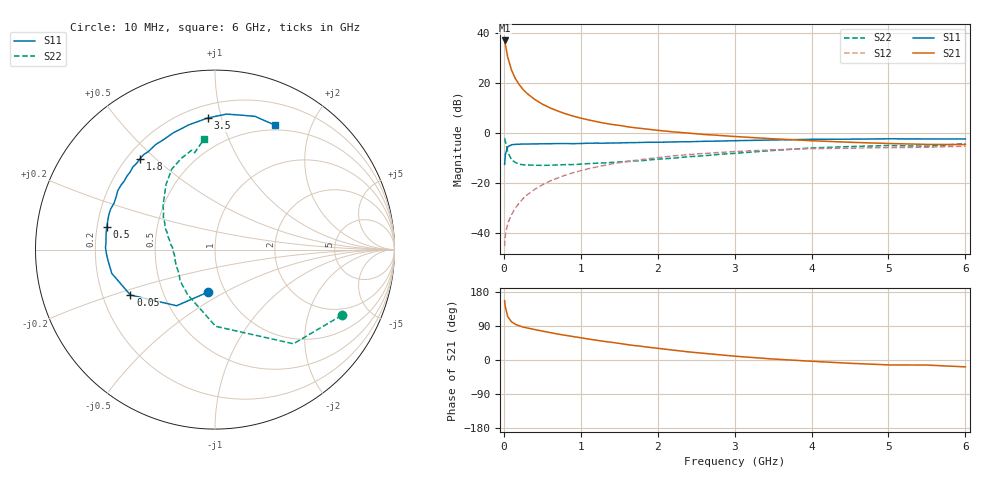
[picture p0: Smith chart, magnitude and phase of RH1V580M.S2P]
! SIEMENS Small Signal Semiconductors
! BFR106
! Si NPN RF Bipolar Junction Transistor in SOT23
! VCE = 1.5 V  IC = 80 mA
! Common Emitter S-Parameters:  August  1996
# GHz  S  MA  R  50
!  f  S11  S21  S12  S22
! GHz  MAG  ANG  MAG  ANG  MAG  ANG  MAG  ANG
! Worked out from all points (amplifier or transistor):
!   36 points, 10 MHz to 6 GHz, reference 50 ohm
!   highest |S21| = 37.2 dB at 10 MHz (marker M1)
!   |S21| within 3 dB of that: start of sweep to 27.98 MHz
!   unconditionally stable (mu >= 1): 141.1 MHz to end of sweep
!   at 250 MHz: K = 1.08, MAG = 20.1 dB, |S12| = -26.1 dB
!   at 1.4 GHz: K = 1.09, MAG = 6.1 dB, |S12| = -12.3 dB
!   at 6 GHz: K = 1.02, MAG = -0.6 dB, |S12| = -5.2 dB
!   S11 on the Smith chart (normalised r, x): 10 MHz: 0.83, -0.42; 50 MHz: 0.32, -0.23; 500 MHz: 0.24, +0.10; 1.8 GHz: 0.25, +0.45; 3.5 GHz: 0.28, +0.91; 6 GHz: 0.44, +1.51
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0.01  0.2388 -98.9  72.15 156.7  0.0055 73.3  0.7956 -27.4
0.02  0.3791 -124.4  59.42 139.6  0.0094 63.6  0.6829 -50.2
0.05  0.535 -151.8  33.65 114.7  0.0156 57.4  0.4275 -89.5
0.1  0.5901 -167.0  18.35 100.7  0.0236 64.0  0.2936 -121.3
0.15  0.5995 -174.3  12.41 94.3  0.0319 67.5  0.2613 -137.9
0.2  0.6055 -177.9  9.421 90.2  0.0404 70.3  0.24 -147.3
0.25  0.6102 178.9  7.528 87.0  0.0494 71.2  0.2345 -155.0
0.3  0.6087 176.4  6.306 84.7  0.058 72.0  0.2325 -159.2
0.4  0.6131 171.9  4.778 80.4  0.0755 72.4  0.2293 -166.3
0.5  0.6157 168.4  3.836 76.3  0.0928 71.8  0.2279 -171.2
0.6  0.6187 164.9  3.226 72.4  0.1107 70.7  0.2292 -174.2
0.7  0.6227 161.8  2.793 68.5  0.1276 69.7  0.2328 -177.0
0.9  0.619 155.3  2.21 61.9  0.1622 66.5  0.2366 177.4
1.1  0.6332 148.9  1.853 55.3  0.1952 63.2  0.2471 173.8
1.4  0.6387 140.4  1.507 46.7  0.2425 57.6  0.2606 167.8
1.8  0.6568 129.4  1.243 35.9  0.2996 50.4  0.2841 160.0
2.2  0.672 119.5  1.068 26.1  0.3515 43.2  0.3173 152.0
2.8  0.6986 105.8  0.907 13.9  0.4133 32.7  0.379 139.8
3.5  0.7347 93.1  0.776 2.6  0.4669 21.5  0.4535 127.0
4.5  0.7629 79.1  0.661 -8.7  0.5041 7.5  0.5421 110.2
5.5  0.7695 68.0  0.599 -13.4  0.5262 -0.8  0.5518 101.9
6  0.77 64.1  0.594 -18.1  0.5502 -7.4  0.6198 95.5
